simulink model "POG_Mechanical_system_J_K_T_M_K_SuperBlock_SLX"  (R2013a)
settings: Solver=ode45  StartTime=0.0  StopTime=10.0  MaxStep=0.001  RelTol=1e-3
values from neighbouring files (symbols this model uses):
  b_1 = 1*Nm/(10*rpm)    (= 0.954929658551)    [POG_Mechanical_system_J_K_T_M_K_Par_SLX_m.m]    (also in POG_Mechanical_system_J_K_T_M_K_SLX_m.m = 1; POG_Mechanical_system_J_K_T_M_K_SuperBlock_SLX_m.m = 1; POG_Mechanical_system_J_K_T_M_K_NL_SLX_m.m)
  J = 1*kg*(30*cm)^2    (= 0.09)    [POG_Mechanical_system_J_K_T_M_K_Par_SLX_m.m]    (also in POG_Mechanical_system_J_K_T_M_K_SLX_m.m = 1; POG_Mechanical_system_J_K_T_M_K_SuperBlock_SLX_m.m = 1; POG_Mechanical_system_J_K_T_M_K_NL_SLX_m.m)
  M = 10*kg    (= 10)    [POG_Mechanical_system_J_K_T_M_K_Par_SLX_m.m]    (also in POG_Mechanical_system_J_K_T_M_K_SLX_m.m = 1; POG_Mechanical_system_J_K_T_M_K_SuperBlock_SLX_m.m = 1; POG_Mass_Linear_Control_SLX_m.m; POG_Mechanical_system_J_K_T_M_K_NL_SLX_m.m)
  P_2_0 = 0    [POG_Mechanical_system_J_K_T_M_K_Par_SLX_m.m]    (also in POG_Mechanical_system_J_K_T_M_K_SLX_m.m; POG_Mechanical_system_J_K_T_M_K_SuperBlock_SLX_m.m; POG_Mechanical_system_J_K_T_M_K_NL_SLX_m.m)
  P_7_0 = 0    [POG_Mechanical_system_J_K_T_M_K_Par_SLX_m.m]    (also in POG_Mechanical_system_J_K_T_M_K_SLX_m.m; POG_Mechanical_system_J_K_T_M_K_SuperBlock_SLX_m.m)
  R = 40*cm    (= 0.4)    [POG_Mechanical_system_J_K_T_M_K_Par_SLX_m.m]    (also in POG_Mechanical_system_J_K_T_M_K_SLX_m.m = 1; POG_Mechanical_system_J_K_T_M_K_SuperBlock_SLX_m.m = 1; POG_Mechanical_system_J_K_T_M_K_NL_SLX_m.m)
  T = 10*Nm    (= 10)    [POG_Mechanical_system_J_K_T_M_K_Par_SLX_m.m]    (also in POG_Mechanical_system_J_K_T_M_K_SLX_m.m; POG_Mechanical_system_J_K_T_M_K_SuperBlock_SLX_m.m; POG_Mechanical_system_J_K_T_M_K_NL_SLX_m.m = 2)
  Ts = Tfin/Nr_Ts_Points    (= 0.0025)    [POG_Mechanical_system_J_K_T_M_K_Par_SLX_m.m]    (also in POG_Mechanical_system_J_K_T_M_K_SLX_m.m = 0.005; POG_Mechanical_system_J_K_T_M_K_SuperBlock_SLX_m.m = 0.005; POG_Mass_Linear_Control_SLX_m.m; POG_Mechanical_system_J_K_T_M_K_NL_SLX_m.m)
  v_d = 0    [POG_Mechanical_system_J_K_T_M_K_Par_SLX_m.m]    (also in POG_Mechanical_system_J_K_T_M_K_SLX_m.m; POG_Mechanical_system_J_K_T_M_K_SuperBlock_SLX_m.m; POG_Mechanical_system_J_K_T_M_K_NL_SLX_m.m)
  x_6_0 = 0    [POG_Mechanical_system_J_K_T_M_K_Par_SLX_m.m]    (also in POG_Mechanical_system_J_K_T_M_K_SLX_m.m; POG_Mechanical_system_J_K_T_M_K_SuperBlock_SLX_m.m; POG_Mechanical_system_J_K_T_M_K_NL_SLX_m.m)
  x_9_0 = 0    [POG_Mechanical_system_J_K_T_M_K_Par_SLX_m.m]    (also in POG_Mechanical_system_J_K_T_M_K_SLX_m.m; POG_Mechanical_system_J_K_T_M_K_SuperBlock_SLX_m.m; POG_Mechanical_system_J_K_T_M_K_NL_SLX_m.m)
undefined symbols (not defined in the file or in its folder): b2, K1, K2

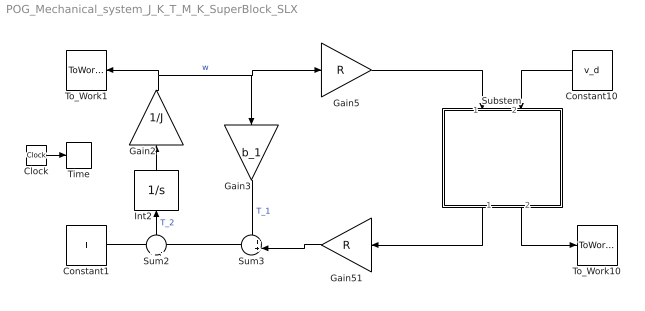
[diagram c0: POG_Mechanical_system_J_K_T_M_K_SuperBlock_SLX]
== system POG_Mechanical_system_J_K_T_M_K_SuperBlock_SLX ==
  Clock : Clock
  Constant1 : Constant  Value=T
  Constant10 : Constant  Value=v_d
  Gain2 : Gain  Gain=1/J
  Gain3 : Gain  Gain=b_1
  Gain5 : Gain  Gain=R
  Gain51 : Gain  Gain=R
  Int2 : Integrator  InitialCondition=P_2_0
  Substem : Subsystem
  Sum2 : Sum  Inputs=+|-
  Sum3 : Sum  Inputs=++|
  Time : ToWorkspace  VariableName=t  SampleTime=Ts
  To_Work1 : ToWorkspace  VariableName=w_1  SampleTime=Ts
  To_Work10 : ToWorkspace  VariableName=F_d  SampleTime=Ts
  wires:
  Constant1/1 -> Sum2/1
  Sum3/1 -> Sum2/2
  Gain2/1 -> To_Work1/1, Gain3/1, Gain5/1  "w"
  Sum2/1 -> Int2/1  "T_2"
  Int2/1 -> Gain2/1
  Gain51/1 -> Sum3/2
  Gain3/1 -> Sum3/1  "T_1"
  Clock/1 -> Time/1
  Gain5/1 -> Substem/1(W_r)
  Constant10/1 -> Substem/2(v_d)
  Substem/1(F_1) -> Gain51/1
  Substem/2(F_2) -> To_Work10/1

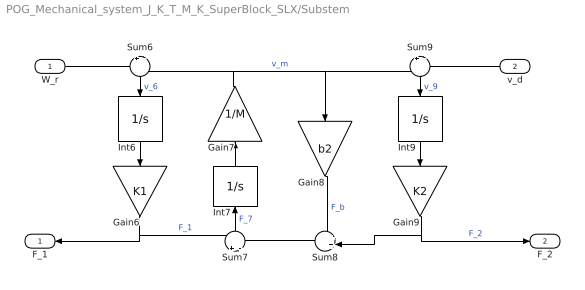
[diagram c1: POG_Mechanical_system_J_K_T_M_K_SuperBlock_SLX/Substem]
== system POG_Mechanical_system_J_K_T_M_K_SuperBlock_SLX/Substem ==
  W_r : Inport
  v_d : Inport  Port=2
  Gain6 : Gain  Gain=K1
  Gain7 : Gain  Gain=1/M
  Gain8 : Gain  Gain=b2
  Gain9 : Gain  Gain=K2
  Int6 : Integrator  InitialCondition=x_6_0
  Int7 : Integrator  InitialCondition=P_7_0
  Int9 : Integrator  InitialCondition=x_9_0
  Sum6 : Sum  Inputs=+|-
  Sum7 : Sum  Inputs=+|-
  Sum8 : Sum  Inputs=++|
  Sum9 : Sum  Inputs=+|-
  F_1 : Outport
  F_2 : Outport  Port=2
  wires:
  Gain9/1 -> F_2/1, Sum8/2  "F_2"
  Sum7/1 -> Int7/1  "F_7"
  W_r/1 -> Sum6/1
  Sum6/1 -> Int6/1  "v_6"
  Gain7/1 -> Sum6/2, Gain8/1, Sum9/1  "v_m"
  Int6/1 -> Gain6/1
  Int9/1 -> Gain9/1
  Sum9/1 -> Int9/1  "v_9"
  v_d/1 -> Sum9/2
  Gain8/1 -> Sum8/1  "F_b"
  Sum8/1 -> Sum7/2
  Gain6/1 -> F_1/1, Sum7/1  "F_1"
  Int7/1 -> Gain7/1
